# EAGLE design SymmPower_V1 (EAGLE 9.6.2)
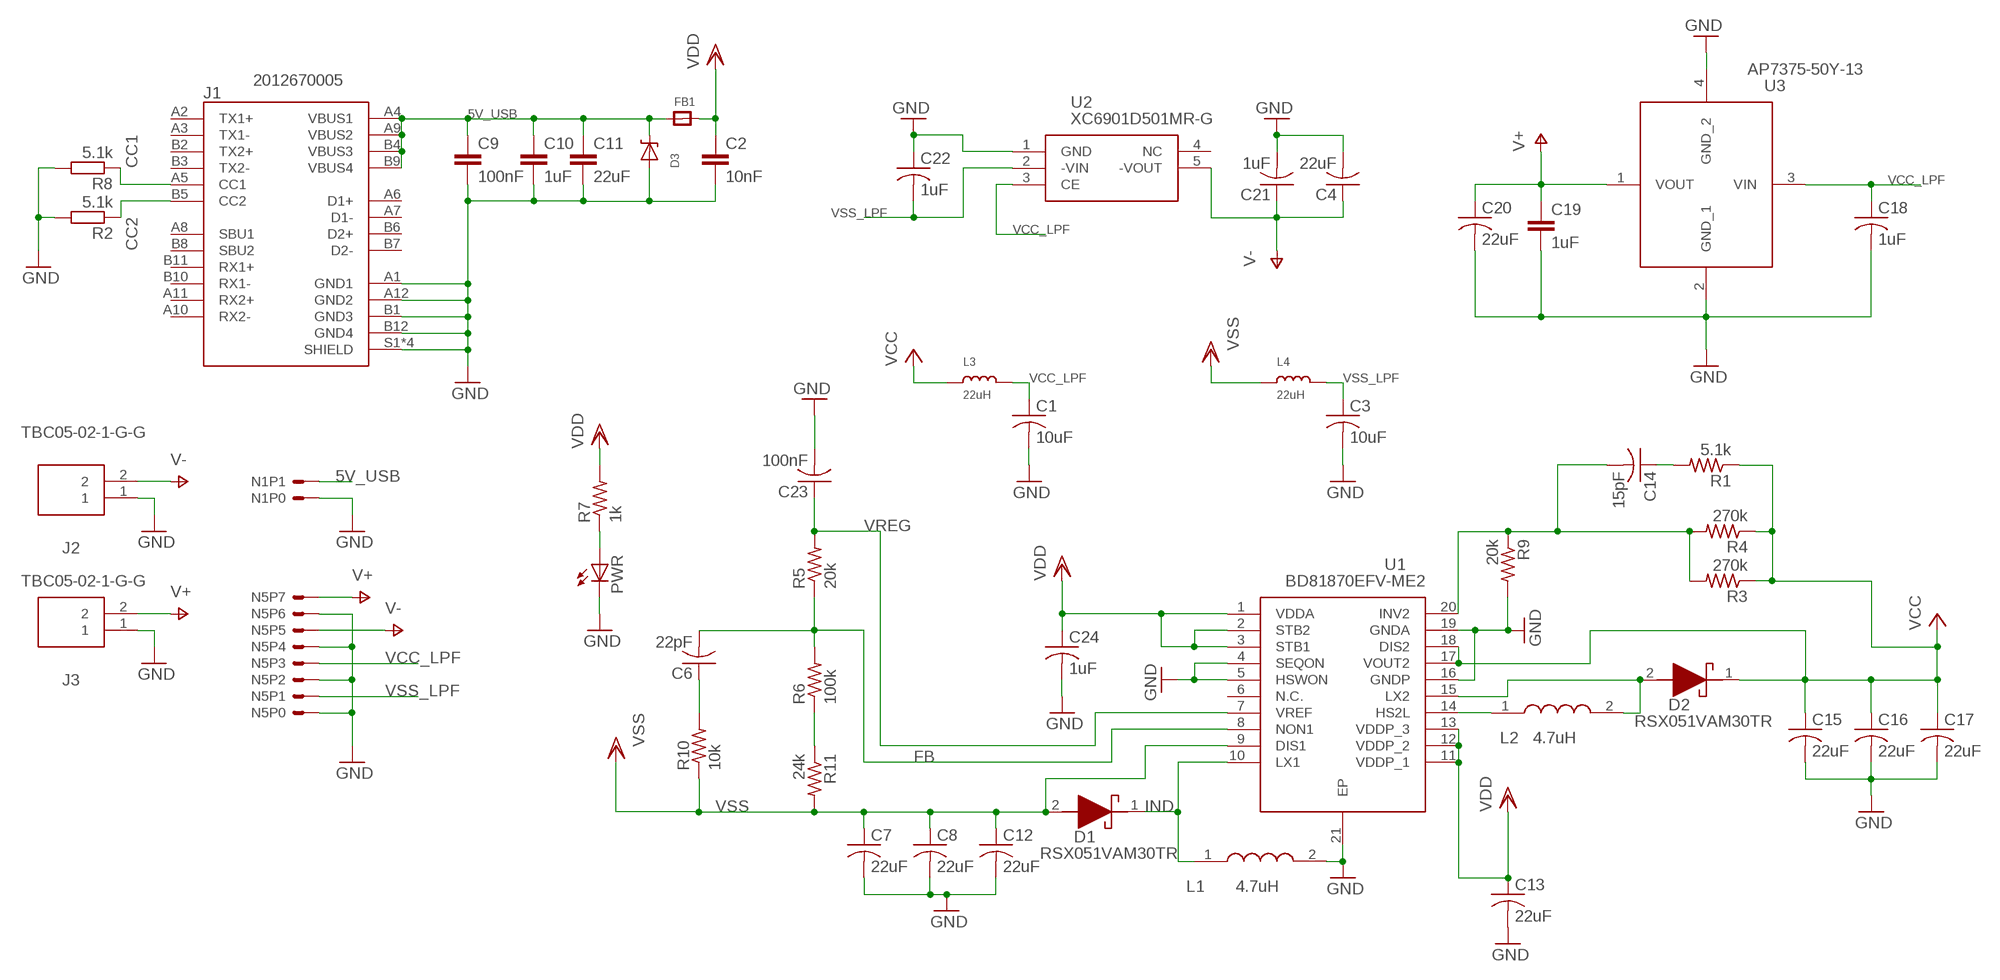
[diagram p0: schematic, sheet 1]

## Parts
C1  10uF  C-USC0603  [C0603]
C2  10nF  C-EUC0603  [C0603]
C3  10uF  C-USC0603  [C0603]
C4  22uF  C-USC0603  [C0603]
C6  22pF  C-USC0603  [C0603]
C7  22uF  C-USC0603  [C0603]
C8  22uF  C-USC0603  [C0603]
C9  100nF  C-EUC0603  [C0603]
C10  1uF  C-EUC0603  [C0603]
C11  22uF  C-EUC0603  [C0603]
C12  22uF  C-USC0603  [C0603]
C13  22uF  C-USC0603  [C0603]
C14  15pF  C-USC0603  [C0603]
C15  22uF  C-USC0603  [C0603]
C16  22uF  C-USC0603  [C0603]
C17  22uF  C-USC0603  [C0603]
C18  1uF  C-USC0603  [C0603]
C19  1uF  C-EUC0603  [C0603]
C20  22uF  C-USC0603  [C0603]
C21  1uF  C-USC0603  [C0603]
C22  1uF  C-USC0603  [C0603]
C23  100nF  C-USC0603  [C0603]
C24  1uF  C-USC0603  [C0603]
D1  RSX051VAM30TR  [RSX051VAM30TR]
D2  RSX051VAM30TR  [RSX051VAM30TR]
D3  DDZ5V6ASF  [DDZ5V6ASF]
FB1  FERRITE_0603  [_0603]
J1  2012670005  [MOLEX_2012670005]
J2  TBC05-02-1-G-G  [TBC05021GG]
J3  TBC05-02-1-G-G  [TBC05021GG]
L1  4.7uH  LQM21PN4R7MGSD  [LQM21PHR47NG0D]
L2  4.7uH  LQM21PN4R7MGSD  [LQM21PHR47NG0D]
L3  22uH  INDUCTOR0805  [0805]
L4  22uH  INDUCTOR0805  [0805]
N1  2PINHEADER  [2PINHEADER]
N5  8PINHEADER  [8PINHEADER]
PWR  LEDCHIPLED_0603  [CHIPLED_0603]
R1  5.1k  R-US_R0603  [R0603]
R2  5.1k  R-EU_R0603  [R0603]
R3  270k  R-US_R0603  [R0603]
R4  270k  R-US_R0603  [R0603]
R5  20k  R-US_R0603  [R0603]
R6  100k  R-US_R0603  [R0603]
R7  1k  R-US_R0603  [R0603]
R8  5.1k  R-EU_R0603  [R0603]
R9  20k  R-US_R0603  [R0603]
R10  10k  R-US_R0603  [R0603]
R11  24k  R-US_R0603  [R0603]
U1  BD81870EFV-ME2  [SOP65P640X100-21N]
U2  XC6901D501MR-G  [SOT95P280X130-5N]
U3  AP7375-50Y-13  [AZ7042RTRG1]

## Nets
5V_USB: C9.1 C10.1 C11.1 D3.P$2(C) FB1.1 J1.A4(VBUS1) J1.A9(VBUS2) J1.B4(VBUS3) J1.B9(VBUS4) N1.P1
CC1: J1.A5(CC1) R8.1
CC2: J1.B5(CC2) R2.1
FB: C6.2 R5.1 R6.2 U1.8(NON1)
GND: C1.2 C2.2 C3.2 C4.2 C7.2 C8.2 C9.2 C10.2 C11.2 C12.2 C13.2 C15.2 C16.2 C17.2 C18.2 C19.2 C20.2 C21.2 C22.1 C23.2 C24.2 D3.P$1(A) J1.A1(GND1) J1.A12(GND2) J1.B1(GND3) J1.B12(GND4) J1.S1(SHIELD) J1.S2(SHIELD) J1.S3(SHIELD) J1.S4(SHIELD) J2.1 J3.1 L1.2 N1.P0 N5.P0 N5.P2 N5.P4 N5.P6 PWR.C R2.2 R8.2 R9.2 U1.4(SEQON) U1.5(HSWON) U1.16(GNDP) U1.19(GNDA) U1.21(EP) U2.1(GND) U3.2(GND_1) U3.4(GND_2)
IND: D1.1(K) L1.1 U1.10(LX1)
N$10: C6.1 R10.2
N$11: R6.1 R11.1
N$12: L2.1 U1.14(HS2L)
N$13: D2.2(A) L2.2 U1.15(LX2)
N$14: C14.2 R3.2 R4.2 R9.1 U1.20(INV2)
N$15: C14.1 R1.2
N$19: PWR.A R7.1
V+: C19.1 C20.1 J3.2 N5.P7 U3.1(VOUT)
V-: C4.1 C21.1 J2.2 N5.P5 U2.5(-VOUT)
VCC: C15.1 C16.1 C17.1 D2.1(K) L3.1 R1.1 R3.1 R4.1 U1.17(VOUT2) U1.18(DIS2)
VCC_LPF: C1.1 C18.1 L3.2 N5.P3 U2.3(CE) U3.3(VIN)
VDD: C2.1 C13.1 C24.1 FB1.2 R7.2 U1.1(VDDA) U1.2(STB2) U1.3(STB1) U1.11(VDDP_1) U1.12(VDDP_2) U1.13(VDDP_3)
VREG: C23.1 R5.2 U1.7(VREF)
VSS: C7.1 C8.1 C12.1 D1.2(A) L4.1 R10.1 R11.2 U1.9(DIS1)
VSS_LPF: C3.1 C22.2 L4.2 N5.P1 U2.2(-VIN)
Unconnected: J1.A2(TX1+) J1.A3(TX1-) J1.A6(D1+) J1.A7(D1-) J1.A8(SBU1) J1.A10(RX2-) J1.A11(RX2+) J1.B2(TX2+) J1.B3(TX2-) J1.B6(D2+) J1.B7(D2-) J1.B8(SBU2) J1.B10(RX1-) J1.B11(RX1+) U1.6(N.C.) U2.4(NC)

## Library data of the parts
C1 C3 C4 C6-C8 C12-C18 C20-C24 = rcl:C-US: CAPACITOR, American symbol; SPICEPREFIX: C
C2 C9-C11 C19 = rcl:C-EU: CAPACITOR, European symbol; SPICEPREFIX: C
D1 D2 = SamacSys_Parts:RSX051VAM30TR: ROHM 30V 500mA, SiC Schottky Diode, 2-Pin SOD-323HE RSX051VAM30TR; DESCRIPTION: ROHM 30V 500mA, SiC Schottky Diode, 2-Pin SOD-323HE RSX051VAM30TR; HEIGHT: 0.8mm; MANUFACTURER_NAME: ROHM Semiconductor; MANUFACTURER_PART_NUMBER: RSX051VAM30TR; MOUSER_PART_NUMBER: 755-RSX051VAM30TR; MOUSER_PRICE-STOCK: https://www.mouser.co.uk/ProductDetail/ROHM-Semiconductor/RSX051VAM30TR?qs=4v%252BiZTmLVHH6gyykIHF0SA%3D%3D
D3 = ForceTronics:DDZ5V6ASF: DDZ5V6ASF 5.42 Zener Diode
FB1 = microbuilder:FERRITE: Ferrite Bead
J1 = 2012670005:2012670005: USB-C (USB TYPE-C) USB 3.1 (USB 3.1 Gen 2, Superspeed+) Receptacle Connector 24 Position Surface Mount, Right Angle; Through Hole Check availability; AVAILABILITY: In Stock; DESCRIPTION: USB-C (USB TYPE-C) USB 3.2 Gen 2 (USB 3.1 Gen 2, Superspeed + (USB 3.1)) Receptacle Connector 24 Position Surface Mount, Right Angle; Through Hole; MF: Molex; MP: 2012670005; PACKAGE: None; PRICE: None; PURCHASE-URL: https://pricing.snapeda.com/search/part/2012670005/?ref=eda
J2 J3 = SamacSys_Parts:TBC05-02-1-G-G: Fixed Terminal Blocks 2w, 2.54mm Pitch Term-Block, Side Entry, TH, Rising Clamp; DESCRIPTION: Fixed Terminal Blocks 2w, 2.54mm Pitch Term-Block, Side Entry, TH, Rising Clamp; HEIGHT: 8.8mm; MANUFACTURER_NAME: GCT (GLOBAL CONNECTOR TECHNOLOGY); MANUFACTURER_PART_NUMBER: TBC05-02-1-G-G
L1 L2 = SamacSys_Parts:LQM21PN4R7MGSD: LQM21PN_GS Series Inductor 4.7uH +/-20% 0805 (2012); DESCRIPTION: LQM21PN_GS Series Inductor 4.7uH +/-20% 0805 (2012); HEIGHT: 1mm; MANUFACTURER_NAME: Murata Electronics; MANUFACTURER_PART_NUMBER: LQM21PN4R7MGSD; MOUSER_PART_NUMBER: 81-LQM21PN4R7MGSD; MOUSER_PRICE-STOCK: https://www.mouser.co.uk/ProductDetail/Murata-Electronics/LQM21PN4R7MGSD?qs=Gufeu08L%2Fl2uzbzo%2FrY4bg%3D%3D
L3 L4 = microbuilder:INDUCTOR: Inductors
N1 = ForceTronics:2PINHEADER
N5 = ForceTronics:8PINHEADER: 8 pin header with 2.54mm spacing
PWR = adafruit:LED: LED
R1 R3-R7 R9-R11 = rcl:R-US_: RESISTOR, American symbol; SPICEPREFIX: R
R2 R8 = rcl:R-EU_: RESISTOR, European symbol; SPICEPREFIX: R
U1 = SamacSys_Parts:BD81870EFV-ME2: ROHM - BD81870EFV-ME2 - DC/DC Switching Regulator, Inverting, Step Up, 2 Output, 2.5V to 5.5VIn, 18V out, 2.1MHz, HTSSOP-20 Source: Datasheet; DESCRIPTION: ROHM - BD81870EFV-ME2 - DC/DC Switching Regulator, Inverting, Step Up, 2 Output, 2.5V to 5.5VIn, 18V out, 2.1MHz, HTSSOP-20; HEIGHT: 1mm; MANUFACTURER_NAME: ROHM Semiconductor; MANUFACTURER_PART_NUMBER: BD81870EFV-ME2; MOUSER_PART_NUMBER: 755-BD81870EFV-ME2; MOUSER_PRICE-STOCK: https://www.mouser.co.uk/ProductDetail/ROHM-Semiconductor/BD81870EFV-ME2/?qs=HXFqYaX1Q2wm5IkeUd4YKg%3D%3D
U2 = SamacSys_Parts:XC6901D501MR-G: LDO Voltage Regulators Source: Datasheet; DESCRIPTION: LDO Voltage Regulators; HEIGHT: 1.3mm; MANUFACTURER_NAME: Torex; MANUFACTURER_PART_NUMBER: XC6901D501MR-G; MOUSER_PART_NUMBER: 865-XC6901D501MR-G; MOUSER_PRICE-STOCK: https://www.mouser.co.uk/ProductDetail/Torex-Semiconductor/XC6901D501MR-G?qs=AsjdqWjXhJ83wf2WZneG3A%3D%3D
U3 = SamacSys_Parts:AP7375-50Y-13: LDO Voltage Regulators LDO CMOS LowCurr SOT89 T&R 2.5K Source: Datasheet; DESCRIPTION: LDO Voltage Regulators LDO CMOS LowCurr SOT89 T&R 2.5K; HEIGHT: 1.6mm; MANUFACTURER_NAME: Diodes Incorporated; MANUFACTURER_PART_NUMBER: AP7375-50Y-13; MOUSER_PART_NUMBER: 621-AP7375-50Y-13; MOUSER_PRICE-STOCK: https://www.mouser.co.uk/ProductDetail/Diodes-Incorporated/AP7375-50Y-13?qs=rQFj71Wb1eXYUkoMPbsPQw%3D%3D

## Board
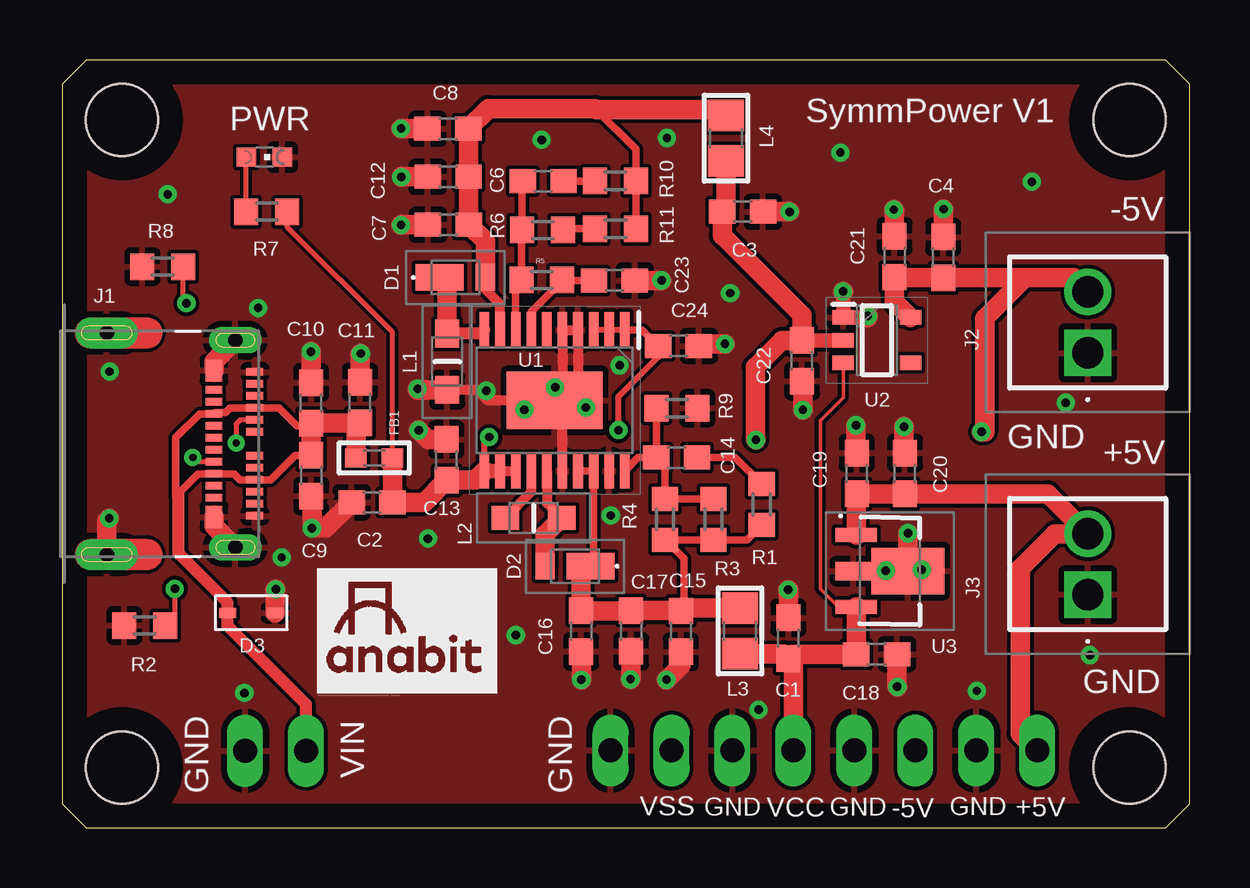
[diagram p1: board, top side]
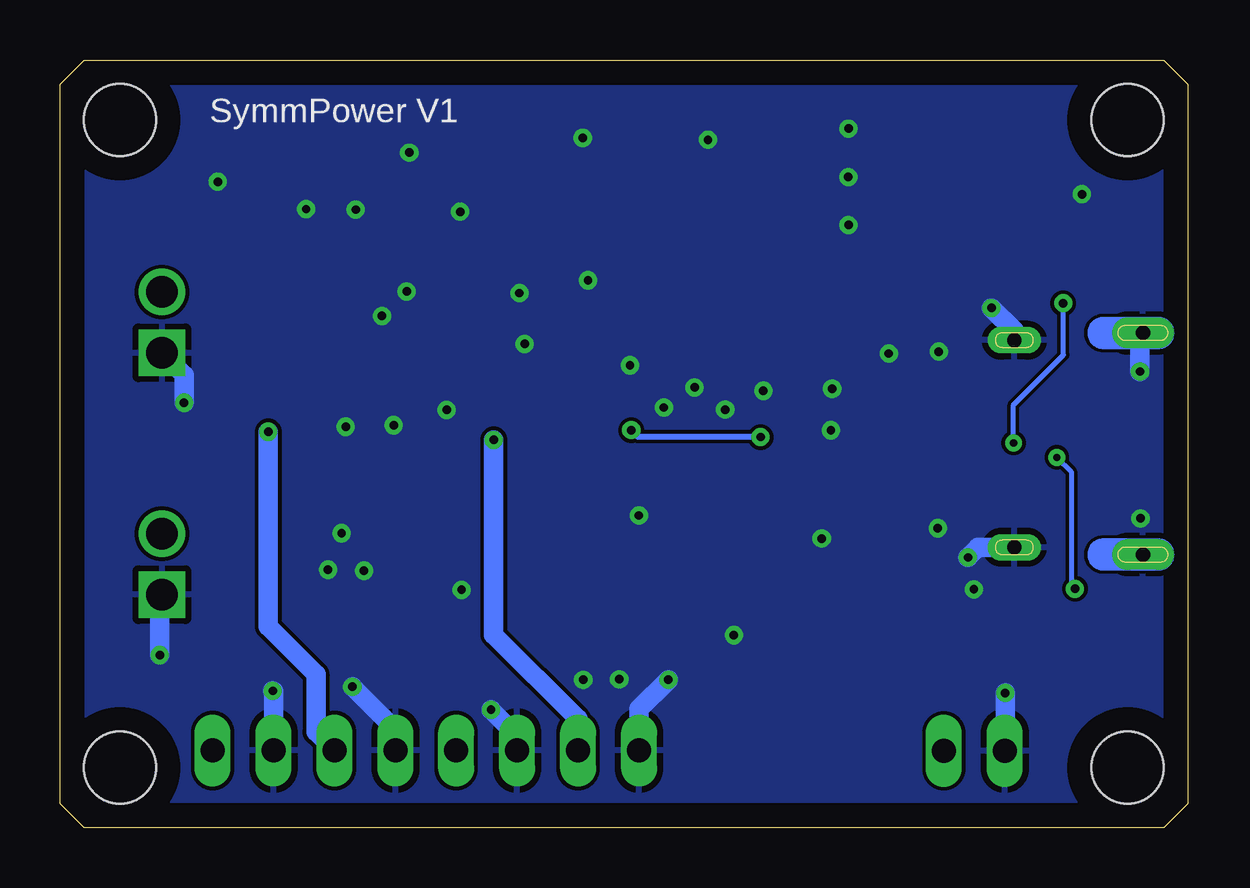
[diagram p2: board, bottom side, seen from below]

Size 47 x 32 mm. Coordinates in mm from the lower left corner, seen from the top.
Outline: 0,31 0,1 1,0 46,0 47,1 47,31 46,32 1,32 0,31
Copper layers (1*16): Top 0.035mm / dielectric 1.5mm / Bottom 0.035mm
Design rules "default *": minimum track width 6mil, minimum drill 0.3mm, track to track 6mil, track to pad 6mil, pad to pad 6mil, via to via 6mil, smd to smd 6mil, copper to edge 40mil, drill to drill 6mil, minimum pad ring 10mil, minimum via ring 8mil, stop-mask expansion 4mil, vias tented up to drill 0mil, thermal gap 10mil
Holes 3 mm at 2.5,2.5 2.5,29.5 44.5,29.5 44.5,2.5

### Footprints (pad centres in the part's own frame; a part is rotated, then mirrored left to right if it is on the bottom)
C0603 = smd 1.1 x 1: 1 -0.85,0; 2 0.85,0
RSX051VAM30TR = smd 1.1 x 2: 1 0,0.65 | smd 1.1 x 0.8: 2 0,-1.25
DDZ5V6ASF = smd 0.71 x 0.41: P$1 0,0; P$2 1.99,0
_0603 = smd 0.9 x 0.8: 1 -0.762,0; 2 0.762,0
MOLEX_2012670005 = smd 0.3 x 0.7: A1 -3,0.81; A2 -2.5,0.81; A3 -2,0.81; A4 -1.5,0.81; A5 -1,0.81; A6 -0.5,0.81; A7 0.5,0.81; A8 1,0.81; A9 1.5,0.81; A10 2,0.81; A11 2.5,0.81; A12 3,0.81; B2 2.25,-0.89; B3 1.75,-0.89; B4 1.25,-0.89; B5 0.75,-0.89; B6 0.25,-0.89; B7 -0.25,-0.89; B8 -0.75,-0.89; B9 -1.25,-0.89; B10 -1.75,-0.89; B11 -2.25,-0.89 | smd 0.9 x 0.7: B1 3.05,-0.89; B12 -3.05,-0.89 | drill 0.6 pad 1.1 long: S1 -4.32,0; S2 4.32,0 | drill 0.6 pad 1.3 long: S3 -4.62,-5.36; S4 4.62,-5.36
TBC05021GG = drill 1.3 pad 1.95 square: 1 0,0 | drill 1.3 pad 1.95: 2 2.54,0
LQM21PHR47NG0D = smd 1.15 x 1: 1 -1.175,0; 2 1.175,0
0805 = smd 1.3 x 1.5: 1 -0.95,0; 2 0.95,0
2PINHEADER = drill 1 long: P0 -1.27,0; P1 1.27,0
8PINHEADER = drill 1 long: P0 1.27,-3.81; P1 3.81,-3.81; P2 6.35,-3.81; P3 8.89,-3.81; P4 11.43,-3.81; P5 13.97,-3.81; P6 16.51,-3.81; P7 19.05,-3.81
CHIPLED_0603 = smd 0.8 x 0.8: A 0,-0.75; C 0,0.75
R0603 = smd 1 x 1.1: 1 -0.85,0; 2 0.85,0
SOP65P640X100-21N = smd 1.475 x 0.4: 1 -2.938,2.925; 2 -2.938,2.275; 3 -2.938,1.625; 4 -2.938,0.975; 5 -2.938,0.325; 6 -2.938,-0.325; 7 -2.938,-0.975; 8 -2.938,-1.625; 9 -2.938,-2.275; 10 -2.938,-2.925; 11 2.938,-2.925; 12 2.938,-2.275; 13 2.938,-1.625; 14 2.938,-0.975; 15 2.938,-0.325; 16 2.938,0.325; 17 2.938,0.975; 18 2.938,1.625; 19 2.938,2.275; 20 2.938,2.925 | smd 2.4 x 4: 21 0,0
SOT95P280X130-5N = smd 0.9 x 0.6: 1 -1.4,0.95; 2 -1.4,0; 3 -1.4,-0.95; 4 1.4,-0.95; 5 1.4,0.95
AZ7042RTRG1 = smd 0.58 x 1.73: 1 -1.5,-1.4; 3 1.5,-1.4 | smd 0.76 x 1.5: 2 0,-1.515 | smd 1.933 x 3.03: 4 0,0.75

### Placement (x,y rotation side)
C1  30.27,7.9 90 top
C2  12.92,13.56 180 top
C3  28.37,25.67 0 top
C4  36.73,23.77 90 top
C6  20.05,26.95 180 top
C7  16.1,25.13 180 top
C8  16.08,29.13 180 top
C9  10.38,14.67 270 top
C10  10.37,17.7 90 top
C11  12.41,17.72 90 top
C12  16.09,27.13 180 top
C13  16.02,15.33 90 top
C14  25.61,15.43 180 top
C15  25.79,8.18 270 top
C16  21.63,8.19 270 top
C17  23.72,8.2 270 top
C18  33.95,7.22 0 top
C19  33.12,14.76 90 top
C20  35.13,14.76 90 top
C21  34.7,23.8 90 top
C22  30.84,19.46 90 top
C23  23.02,22.81 0 top
C24  25.69,20.08 0 top
D1  16.39,22.93 90 top
D2  21.38,10.89 270 top
D3  8.88,8.96 180 top
FB1  13.01,15.41 0 top
J1  7.22,16 270 top
J2  42.75,19.79 90 top
J3  42.75,9.71 90 top
L1  16.05,19.42 270 top
L2  19.65,12.91 0 top
L3  28.25,8.2 270 top
L4  27.67,28.74 270 top
N1  8.89,3.2 0 top
N5  21.59,7.02 0 top
PWR  8.43,27.95 270 top
R1  29.16,13.47 90 top
R2  3.44,8.42 180 top
R3  27.15,12.85 90 top
R4  25.13,12.85 90 top
R5  19.99,22.83 0 top
R6  20.03,24.91 180 top
R7  8.53,25.67 0 top
R8  4.19,23.38 180 top
R9  25.63,17.48 0 top
R10  23.06,26.96 180 top
R11  23.07,24.96 0 top
U1  20.53,17.81 270 top
U2  33.96,20.32 0 top
U3  34.5,10.69 270 top

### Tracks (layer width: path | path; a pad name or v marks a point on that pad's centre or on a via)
5V_USB
  Top 0.305: C10.1 10.27,16.75 9.8,16.75 9.05,17.5 J1.A4 7.01,17.5 6.81,17.3 6.38,17.3 J1.B9 5.73,17.25 4.74,16.26 4.74,13.81 4.85,13.92 5.68,14.75 J1.B4 7.18,14.75 7.43,14.5 J1.A9 8.7,14.5 9.72,15.52 C9.1
  Top 0.508: N1.P1 10.16,5.14 6.89,8.41 D3.P$2 6.89,9.38 4.85,11.42 4.85,13.92
  Top 0.813: C9.1 C10.1 10.39,16.87 C11.1 12.25,16.71 FB1.1
CC1  (via drill 0.3, 0.35)
  Top 0.2: J1.A5 7.43,17 7.25,16.82 v7.25,16.03 | v5.18,21.86 5.04,22 R8.1
  Bottom 0.2: v7.25,16.03 7.25,17.62 5.17,19.7 v5.17,21.86 v5.18,21.86
CC2  (via drill 0.3, 0.35)
  Top 0.2: J1.B5 5.61,15.25 5.45,15.41 v5.45,15.43 | v4.7,9.96 4.7,8.82 R2.1
  Bottom 0.2: v5.45,15.43 4.85,14.83 4.85,10.02 4.74,9.91 v4.7,9.96
FB
  Top 0.305: U1.8 18.91,22.59 R5.1 19.14,24.87 R6.2 19.18,26.93 C6.2
GND  (via drill 0.35)
  Top 0.406: U1.16 20.86,18.05 v20.55,18.35 20.86,18.66 U1.5 U1.4 21.5,17.84 v21.83,17.51 | U1.21 17.74,17.81 17.3,18.25 L1.2
  Top 0.61: v32.56,22.34 U2.1 33.57,21.27
  Top 0.813: C10.2 v10.37,19.84 | C11.2 12.41,19.72 v12.45,19.76 | L1.2 14.81,18.25 v14.81,18.29 | C13.2 15.25,16.18 v14.87,16.57 | D3.P$1 8.88,9.9 v8.9,9.93 | C9.2 10.41,13.79 v10.41,12.48 10.99,12.48 C2.2 | C16.2 v21.64,6.16 | C17.2 23.72,6.21 v23.69,6.18 | C15.2 25.79,6.76 v25.19,6.16 | C1.2 v30.27,9.9 v30.26,9.91 | v34.81,5.87 v34.8,5.88 C18.2 | v35.26,12.27 v35.25,12.26 U3.4 | C24.2 26.62,20.16 v27.63,20.16 | C22.1 30.88,18.57 v30.88,17.41 | C19.2 33.09,15.64 v33.09,16.77 | C20.2 35.09,15.65 v35.09,16.71 | v32.56,22.34 v32.55,22.35 | v33.58,21.33 33.58,21.28 33.57,21.27 | C3.2 v30.32,25.67 | C23.2 v24.99,22.81 | C21.2 34.7,25.73 v34.67,25.76 | C4.2 v36.73,25.77 v36.74,25.78 | C8.2 v14.14,29.13 v14.13,29.14 | C12.2 v14.15,27.13 v14.14,27.12 | C7.2 v14.14,25.13 v14.13,25.12 | J1.B12 6.33,19.43 J1.S1 | J1.B1 6.33,12.57 J1.S2 | J1.S4 1.86,12.79 v1.96,12.89
  Bottom 0.813: N5.P4 33.02,4.08 v34.81,5.87 | N5.P6 38.1,5.67 v38.13,5.7 | J3.1 42.84,9.62 v42.84,7.19 | J2.1 41.83,18.87 v41.83,17.71 | J1.S2 8.73,11.68 v9.15,11.26 | J1.S1 7.22,20.71 v8.17,21.66 | J1.S3 1.98,20.5 v1.98,19.01 | N5.P0 22.86,4.94 v21.64,6.16 | N5.P2 27.94,3.82 v29.03,4.91 | N1.P0 7.6,3.22 v7.6,5.61
  other vias: 4.4,26.4 19.27,17.42 34.33,10.71 15.25,12.05 27.85,22.28 32.44,28.14 40.42,26.92 35.83,10.75 18.91,8.02 19.99,28.67 22.87,13.01 25.21,28.75 23.24,19.27 17.68,18.21
  pour Bottom: -4,34 51,34 51,-2 -4,-2
  pour Top: -2,33 48,33 48,-1 -1,-1 -2,0
IND
  Top 0.508: U1.10 17.45,20.59 L1.1
  Top 0.813: D1.1 16.05,22.62 L1.1
N$10
  Top 0.305: C6.1 R10.2
N$11
  Top 0.305: R6.1 20.93,24.96 R11.1
N$12
  Top 0.406: U1.14 19.55,13.99 L2.1
N$13
  Top 0.406: U1.15 20.2,13.53 L2.2
  Top 0.813: L2.2 20.13,12.21 D2.2
N$14
  Top 0.305: U1.20 24.01,15.43 C14.2 | C14.2 24.78,15.45 R9.1 | C14.2 25.13,15.06 R4.2 R3.2
N$15
  Top 0.305: C14.1 28.05,15.43 R1.2
N$19
  Top 0.2: R7.1 PWR.A
V+
  Top 0.813: U3.1 33.1,13.89 C19.1 C20.1 41.09,13.91 J3.2 41.38,12.25 39.94,10.81 39.94,3.91 N5.P7
V-  (via drill 0.35)
  Top 0.813: U2.5 34.7,21.93 C21.1 34.73,22.92 C4.1 40.15,22.92 | 40.15,22.92 42.16,22.92 J2.2 | 40.15,22.92 38.46,21.23 38.46,16.5 v38.32,16.5
  Bottom 0.813: v38.32,16.5 38.32,8.38 36.33,6.39 36.33,3.98 N5.P5
VCC
  Top 0.305: R1.1 28.54,12 R3.1 R4.1 25.91,11.22 25.91,9.15 | U1.17 U1.18 22.16,11.02 D2.1
  Top 0.813: D2.1 21.63,10.49 C16.1 C17.1 25.77,9.05 C15.1 25.91,9.15 L3.1
VCC_LPF
  Top 0.152: U3.3 32.36,9.19 31.6,9.95 31.6,16.97 32.56,17.93 U2.3
  Top 0.813: L3.2 30.07,7.25 C1.1 | C1.1 30.48,6.84 N5.P3 | C1.1 30.44,7.22 C18.1 U3.3
VDD  (via drill 0.35)
  Top 0.2: FB1.2 13.77,20.65 9.38,25.04 R7.2
  Top 0.254: C24.1 24.84,19.61 23.19,17.96 v23.19,16.57 | U1.11 17.61,16.09 v17.8,16.28 | U1.1 U1.2 U1.3
  Top 0.305: U1.1 24.17,20.75 C24.1
  Top 0.406: U1.12 U1.13
  Top 0.61: U1.11 U1.12
  Top 0.813: FB1.2 C2.1 15.1,13.56 C13.1 17.21,14.48 U1.11
  Bottom 0.254: v23.19,16.57 22.92,16.3 17.82,16.3 v17.8,16.28
VREG
  Top 0.305: U1.7 19.55,21.5 20.84,22.78 R5.2 20.86,22.81 C23.1
VSS
  Top 0.305: R11.2 R10.1 23.91,28.28 22.26,29.93 22.22,29.97
  Top 0.406: U1.9 18.25,21.82 17.64,22.43 D1.2
  Top 0.813: D1.2 17.64,24.44 C7.1 C12.1 C8.1 17.77,29.97 22.22,29.97 | L4.1 27.43,29.93 22.26,29.93
VSS_LPF  (via drill 0.35)
  Top 0.61: C22.2 U2.2
  Top 0.813: L4.2 27.67,25.82 C3.1 27.52,24.68 30.84,21.36 C22.2 30,20.31 28.89,19.2 28.89,16.19 v28.92,16.16
  Bottom 0.813: v28.92,16.16 28.92,8.04 25.41,4.53 N5.P1

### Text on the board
tNames: SymmPower V1 | -5V | GND | +5V | GND | GND | C:/Users/neilf/Dropbox/Anabit/CompanyMessagingBrandingGraphics/Anabit Logo Vertical - Black.bmp | GND | VIN | VSS | GND | GND | VCC | GND | -5V | +5V
bNames: SymmPower V1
